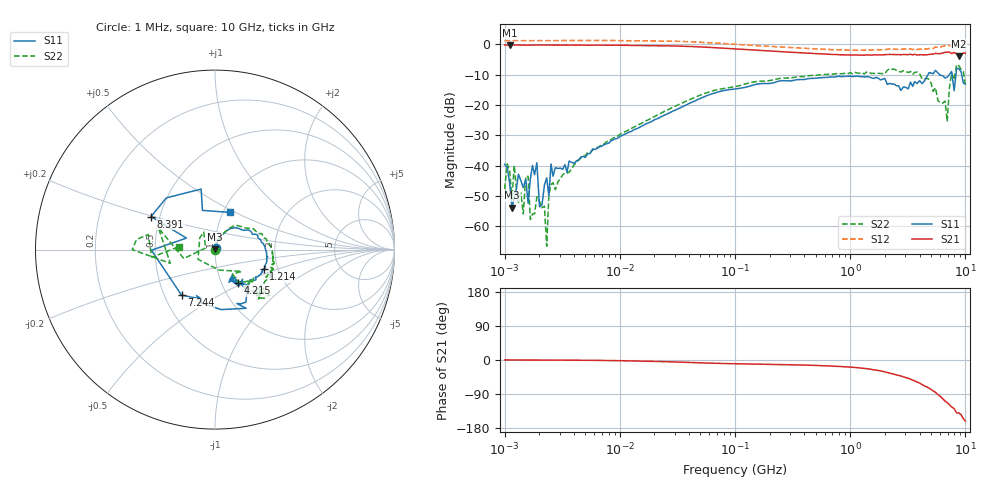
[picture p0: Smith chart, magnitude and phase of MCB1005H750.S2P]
!Agilent Technologies,E5071C,MY46111244,A.11.31
!Date: Tue May 07 16:34:10 2019
!Data & Calibration Information:
!Freq	S11:SOLT2(ON)	S21:SOLT2(ON)	S12:SOLT2(ON)	S22:SOLT2(ON)
# Hz S dB R 50
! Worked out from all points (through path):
!   201 points, 1 MHz to 10 GHz, reference 50 ohm
!   highest |S21| = -0.28 dB at 1.106 MHz (marker M1); lowest = -4.0 dB at 8.793 GHz (marker M2)
!   group delay of S21, straight-line fit = 42.5 ps
!   lowest |S11| = -53.8 dB at 1.159 MHz (marker M3), VSWR 1.00, Z = 50 + j0.198 ohm
!   |S11| at or under -10 dB: start of sweep to 4.738 GHz; 5.976 GHz to 7.256 GHz (1.28 GHz wide, 19.4 % of centre); 9.283 GHz to end of sweep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
!   |S22| runs from -66.5 to -6.7 dB; largest |S21 - S12| = 0.51
!   S11 on the Smith chart (normalised r, x): 1 MHz: 1.01, +0.02; 1.214 GHz: 1.69, -0.40; 4.215 GHz: 1.19, -0.46; 7.244 GHz: 0.61, -0.34; 8.391 GHz: 0.45, +0.20; 10 GHz: 1.07, +0.47
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1000000  -39.56 48.9  -0.30 -0.0  1.14 -0.8  -47.65 -59.7
1106086  -45.68 149.2  -0.28 -0.0  1.13 -0.8  -41.66 -67.1
1159128  -53.80 103.3  -0.29 0.0  1.16 -0.7  -51.04 -56.2
1212171  -50.62 -132.2  -0.30 0.1  1.16 -0.8  -39.89 -37.3
1318257  -42.80 53.6  -0.30 0.0  1.16 -0.9  -52.05 -20.9
1600043  -52.31 150.8  -0.33 -0.1  1.11 -0.5  -43.53 -38.8
1673262  -44.36 58.7  -0.30 -0.1  1.16 -0.9  -57.70 5.5
2216092  -46.38 80.9  -0.33 -0.2  1.18 -1.2  -53.31 50.3
2319636  -44.00 75.1  -0.31 -0.2  1.18 -1.0  -66.48 48.1
2526724  -39.42 76.0  -0.32 -0.3  1.16 -1.0  -46.31 83.9
4810209  -36.95 84.3  -0.33 -0.7  1.17 -1.4  -36.94 77.9
2.206931e7  -24.22 69.4  -0.51 -4.0  1.05 -4.3  -23.02 68.9
1.047129e8  -14.66 36.7  -1.62 -10.0  -0.07 -10.0  -13.83 37.3
4.810209e8  -11.27 5.3  -3.09 -14.3  -1.53 -13.0  -10.29 4.9
1.213756e9  -10.67 -21.8  -3.60 -20.9  -2.00 -17.9  -9.51 -24.1
2.206931e9  -12.91 -52.5  -3.38 -34.6  -1.59 -28.6  -8.02 -39.9
4.215088e9  -13.01 -55.7  -3.48 -65.0  -1.57 -54.5  -11.52 -50.4
6.952868e9  -10.88 -105.0  -2.66 -112.6  -0.57 -95.0  -25.45 170.1
7.24436e9  -10.04 -126.3  -2.62 -117.5  -0.41 -99.3  -14.86 -164.0
8.390517e9  -7.93 152.7  -3.17 -139.7  -0.60 -120.3  -6.72 -180.0
8.792888e9  -8.05 133.2  -3.96 -139.8  -0.18 -121.8  -7.12 172.6
1e10  -13.05 68.6  -3.03 -161.2  0.91 -141.0  -13.93 175.3
